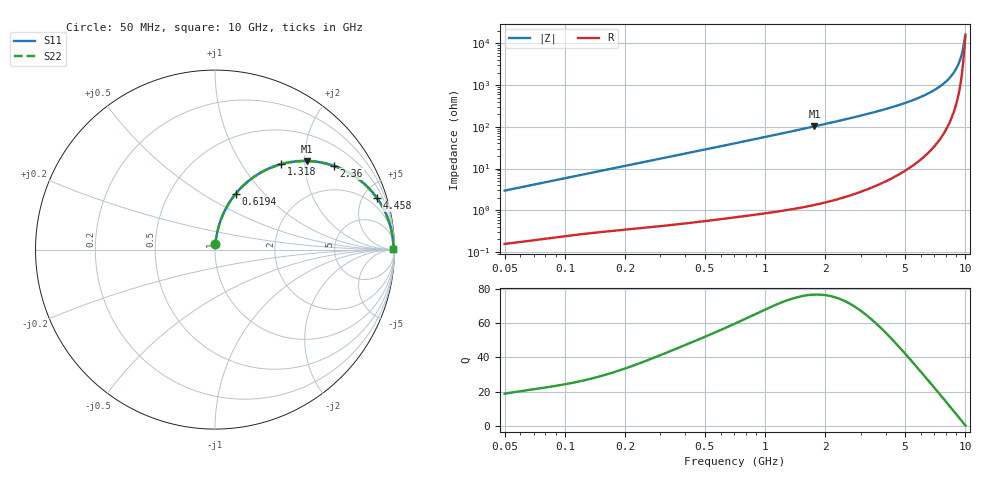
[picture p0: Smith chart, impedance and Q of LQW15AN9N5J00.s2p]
!Murata Part Number: LQW15AN9N5J00
!These Parameters are Measured in Series Mode Connection
!  o--[Z]--o
!Port1  Port2
!  o-------o
!Freq. Start=50[MHz] Stop=10[GHz], 401[Steps]
# Hz S RI R 50
!Freq.(Hz)	S 11(Real)	S 11(Imag)	S 21(Real)	S 21(Imag)	S 12(Real)	S 12(Imag)	S 22(Real)	S 22(Imag)
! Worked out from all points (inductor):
!   401 points, 50 MHz to 10 GHz, reference 50 ohm
!   read as one part in series: L = 9.38 nH near 51.34 MHz
!   highest Q = 76.6 at 1.764 GHz (marker M1), where L = 9.29 nH
!   S11 on the Smith chart (normalised r, x): 50 MHz: 1.00, +0.06; 619.4 MHz: 1.01, +0.71; 1.318 GHz: 1.02, +1.52; 2.36 GHz: 1.04, +2.82; 4.458 GHz: 1.13, +6.26; 10 GHz: open
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5e7  0.00243 0.0295  0.9976 -0.0295  0.9976 -0.0295  0.00243 0.0295
1.214486e8  0.00759 0.0699  0.9924 -0.0699  0.9924 -0.0699  0.00759 0.0699
2.949953e8  0.0316 0.1631  0.9684 -0.1631  0.9684 -0.1631  0.0316 0.1631
6.19383e8  0.1155 0.3109  0.8845 -0.3109  0.8845 -0.3109  0.1155 0.3109
7.071068e8  0.1444 0.3432  0.8556 -0.3432  0.8556 -0.3432  0.1444 0.3432
9.589462e8  0.2348 0.4165  0.7652 -0.4165  0.7652 -0.4165  0.2348 0.4165
1.31782e9  0.3674 0.4753  0.6326 -0.4753  0.6326 -0.4753  0.3674 0.4753
1.717543e9  0.5003 0.4935  0.4997 -0.4935  0.4997 -0.4935  0.5003 0.4935
1.763651e9  0.5142 0.4933  0.4858 -0.4933  0.4858 -0.4933  0.5142 0.4933
2.360312e9  0.6638 0.4657  0.3362 -0.4657  0.3362 -0.4657  0.6638 0.4657
3.158828e9  0.7931 0.3975  0.2069 -0.3975  0.2069 -0.3975  0.7931 0.3975
4.171863e9  0.8854 0.3091  0.1146 -0.3091  0.1146 -0.3091  0.8854 0.3091
4.457516e9  0.9027 0.2863  0.0973 -0.2863  0.0973 -0.2863  0.9027 0.2863
5.437278e9  0.9443 0.2164  0.0557 -0.2164  0.0557 -0.2164  0.9443 0.2164
6.374006e9  0.9676 0.1601  0.0324 -0.1601  0.0324 -0.1601  0.9676 0.1601
7.276762e9  0.9811 0.1133  0.0189 -0.1133  0.0189 -0.1133  0.9811 0.1133
8.090191e9  0.9884 0.0762  0.0116 -0.0762  0.0116 -0.0762  0.9884 0.0762
8.759398e9  0.992 0.0485  0.008 -0.0485  0.008 -0.0485  0.992 0.0485
9.236013e9  0.9935 0.03  0.00651 -0.03  0.00651 -0.03  0.9935 0.03
9.48396e9  0.994 0.0208  0.00602 -0.0208  0.00602 -0.0208  0.994 0.0208
9.868415e9  0.9944 0.00696  0.00562 -0.00696  0.00562 -0.00696  0.9944 0.00696
1e10  0.9944 0.00235  0.00557 -0.00235  0.00557 -0.00235  0.9944 0.00235
